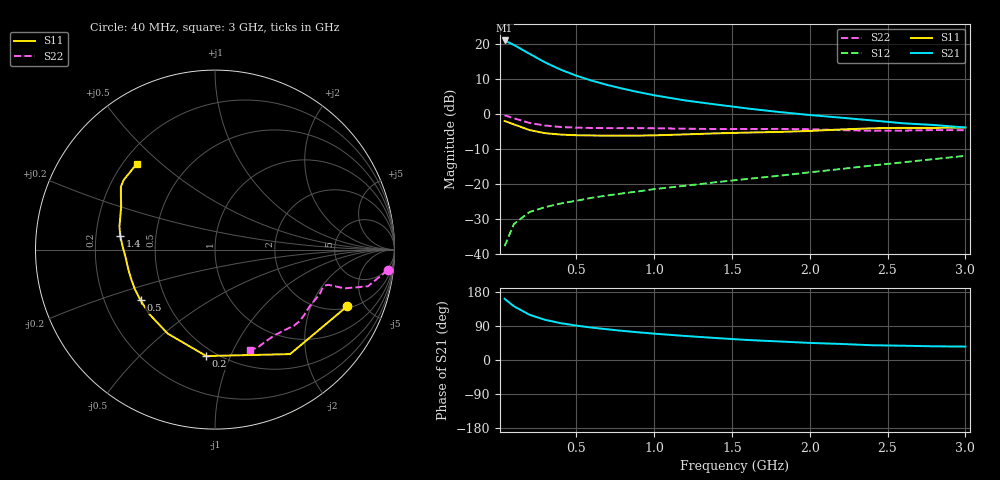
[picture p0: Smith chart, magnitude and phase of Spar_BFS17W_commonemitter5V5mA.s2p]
! Filename:  BFS17WB.S2P  Version:  4.0
! NXP part #: BFS17W  Date: Jun 1994
! Bias condition: Vce=5V, Ic=5mA
#  MHz  S  MA  R  50
! Freq  S11  S21  S12  S22  !GUM [dB]
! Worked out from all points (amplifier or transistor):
!   21 points, 40 MHz to 3 GHz, reference 50 ohm
!   highest |S21| = 21.1 dB at 40 MHz (marker M1)
!   |S21| within 3 dB of that: start of sweep to 167.7 MHz
!   unconditionally stable (mu >= 1): 556.6 MHz to end of sweep
!   at 300 MHz: K = 0.70, MSG = 20.7 dB, |S12| = -26.6 dB
!   at 1 GHz: K = 1.21, MAG = 10.6 dB, |S12| = -21.4 dB
!   at 3 GHz: K = 1.04, MAG = 2.9 dB, |S12| = -11.9 dB
!   S11 on the Smith chart (normalised r, x): 40 MHz: 2.13, -3.75; 200 MHz: 0.45, -0.82; 500 MHz: 0.36, -0.27; 1.4 GHz: 0.31, +0.07; 3 GHz: 0.25, +0.42
40  0.802 -23.1  11.38 161.5  0.013 77.1  0.969 -6.8
100  0.717 -54.3  9.802 141.7  0.027 62.7  0.876 -13.5
200  0.595 -94.7  7.337 119.3  0.04 52.5  0.752 -16.7
300  0.537 -119.4  5.526 106.0  0.047 50.1  0.691 -17.0
400  0.513 -135.2  4.353 97.2  0.053 51.2  0.659 -17.3
500  0.502 -145.7  3.569 90.8  0.058 52.9  0.644 -18.2
600  0.498 -153.7  3.029 85.5  0.064 55.4  0.637 -19.3
700  0.495 -160.1  2.626 81.0  0.069 57.5  0.635 -20.4
800  0.495 -165.6  2.323 76.8  0.074 59.7  0.635 -21.5
900  0.496 -170.4  2.075 73.0  0.079 61.8  0.634 -22.7
1000  0.5 -174.9  1.875 69.6  0.085 63.6  0.632 -23.9
1200  0.516 177.6  1.579 63.4  0.095 67.3  0.622 -27.1
1400  0.534 171.6  1.379 57.9  0.107 71.0  0.615 -31.3
1600  0.548 166.3  1.212 52.8  0.119 74.3  0.616 -36.1
1800  0.559 160.6  1.081 49.0  0.132 77.9  0.618 -40.0
2000  0.578 154.7  0.977 45.1  0.148 80.9  0.611 -44.0
2200  0.607 149.8  0.895 42.4  0.165 83.4  0.594 -48.7
2400  0.631 146.2  0.817 38.9  0.185 85.4  0.581 -55.1
2600  0.64 142.6  0.744 37.7  0.206 86.4  0.585 -61.5
2800  0.64 138.1  0.702 36.1  0.229 87.3  0.595 -66.6
3000  0.647 132.5  0.648 35.4  0.255 87.7  0.593 -70.6
